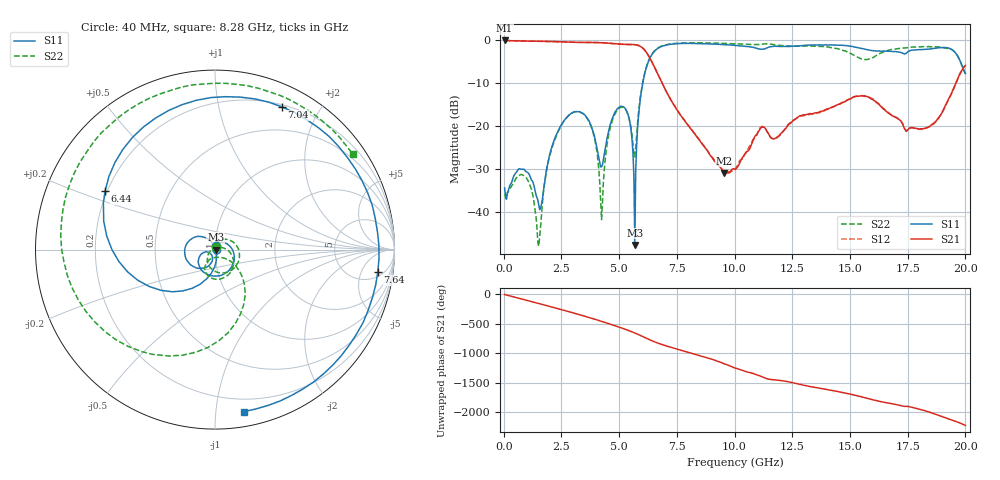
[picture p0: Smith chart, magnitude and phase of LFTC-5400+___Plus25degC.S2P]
! Mini-Circuits
! S2P DATA File Format
! Type: Low Pass LTCC Surface Mount Filter
! Model: LFTC-5400+
! Note: All S Parameters are in dB deg format
! TEST CONDITIONS: INPUT POWER = 0dBm @Temperature = +25degC
! 401 Frequency points
# MHz S DB R 50
!  FREQ  dB(S11)  PHS(S11)  dB(S21)  PHS(S21)  dB(S12)  PHS(S12)  dB(S22)  PHS(S22)
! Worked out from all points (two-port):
!   401 points, 40 MHz to 20 GHz, reference 50 ohm
!   highest |S21| = -0.06 dB at 40 MHz (marker M1); lowest = -30.9 dB at 9.56 GHz (marker M2)
!   |S21| within 3 dB of the highest: start of sweep to 6.211 GHz
!   lowest |S11| = -47.6 dB at 5.68 GHz (marker M3), VSWR 1.01, Z = 50.4 + j0.024 ohm
!   |S11| at or under -10 dB: start of sweep to 6.023 GHz
!   |S22| runs from -47.9 to -0.6 dB; largest |S21 - S12| = 0.0068
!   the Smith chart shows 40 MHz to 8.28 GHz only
!   S11 on the Smith chart (normalised r, x): 40 MHz: 1.01, +0.04; 6.44 GHz: 0.19, +0.24; 7.04 GHz: 0.22, +1.55; 7.64 GHz: 7, -10; 8.28 GHz: 0.10, -1.19
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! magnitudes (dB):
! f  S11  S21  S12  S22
! 40 MHz  -34.4  -0.1  -0.1  -35.8
! 960 MHz  -30.6  -0.2  -0.2  -32.0
! 1.52 GHz  -38.4  -0.2  -0.2  -47.9
! 2.16 GHz  -23.7  -0.3  -0.3  -23.9
! 3.4 GHz  -16.9  -0.5  -0.5  -16.9
! 3.92 GHz  -22.1  -0.5  -0.5  -22.5
! 4.24 GHz  -29.4  -0.6  -0.6  -41.7
! 4.6 GHz  -19.9  -0.7  -0.7  -20.7
! 5.16 GHz  -15.4  -0.9  -1.0  -15.6
! 5.68 GHz  -47.6  -1.0  -1.0  -27.1
! 5.96 GHz  -12.0  -1.6  -1.6  -11.7
! 6.44 GHz  -3.2  -5.3  -5.2  -3.1
! 6.72 GHz  -1.8  -8.4  -8.4  -1.7
! 7.04 GHz  -1.1  -11.9  -11.9  -1.0
! 7.64 GHz  -0.8  -17.2  -17.2  -0.7
! 8.28 GHz  -0.8  -21.8  -21.8  -0.6
! 9.56 GHz  -1.0  -30.9  -30.5  -0.7
! 10.04 GHz  -1.2  -30.1  -29.8  -0.8
! 13.36 GHz  -1.1  -17.1  -17.2  -1.3
! 16.72 GHz  -2.6  -17.1  -17.1  -2.3
! 18.48 GHz  -2.0  -19.9  -20.0  -1.5
! 20 GHz  -7.7  -5.8  -5.9  -7.8
